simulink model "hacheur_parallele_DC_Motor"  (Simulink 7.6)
settings: Solver=ode23tb  StartTime=0.0  StopTime=500  RelTol=1e-3
InitFcn:
  | clc
  | R1=1e3;
  | R2=1e3;
StopFcn:
  | clc
  | close all
  | load vit_pos.mat
  | plotyy(x(1,:),x(2,:),x(1,:),x(3,:))
  | xlabel('temps')
  | title('position et vitesse de rotation')
  | grid
  | 
  | figure
  | 
  | load Us_CdePWM.mat
  | plotyy(y(1,:),y(2,:),y(1,:),y(3,:))
  | xlabel('temps')
  | title('Entrée PWM et tension de sortie du hâcheur parallèle')
  | grid
  | 
  | delete *.mat
libraries: fl_lib x23, powerlib x11, nesl_utility x10, elec_lib x5

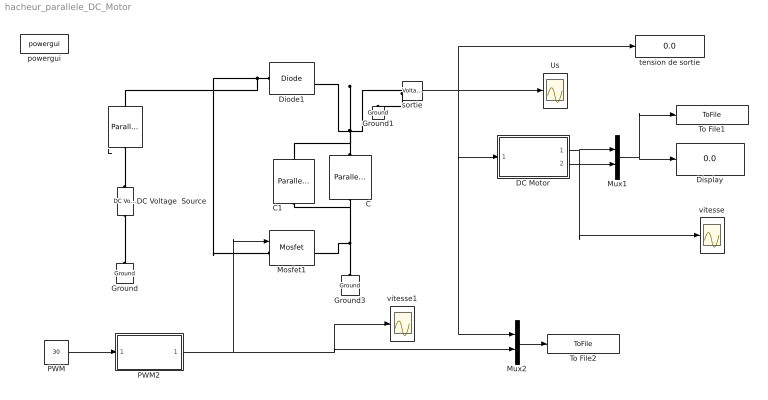
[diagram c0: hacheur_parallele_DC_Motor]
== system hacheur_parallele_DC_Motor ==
  C : powerlib/Elements/Parallel RLC Branch  DialogController=POWERSYS.PowerSysDialog  PhysicalDomain=powersysdomain  SubClassName=unknown  LeftPortType=p1  RightPortType=p1  LConnTagsString=a  RConnTagsString=__new0  BranchType=C  Resistance=1  Inductance=1e-3  SetiL0=off  InitialCurrent=0  Capacitance=1  Setx0=off  InitialVoltage=0  Measurements=None
  C1 : powerlib/Elements/Parallel RLC Branch  DialogController=POWERSYS.PowerSysDialog  PhysicalDomain=powersysdomain  SubClassName=unknown  LeftPortType=p1  RightPortType=p1  LConnTagsString=a  RConnTagsString=__new0  BranchType=C  Resistance=1  Inductance=1e-3  SetiL0=off  InitialCurrent=0  Capacitance=1  Setx0=off  InitialVoltage=0  Measurements=None
  DC Motor : Subsystem
  DC Voltage  Source : powerlib/Electrical Sources/DC Voltage Source  DialogController=POWERSYS.PowerSysDialog  SystemSampleTime=-1  Amplitude=12  Measurements=None
  Diode1 : powerlib/Power Electronics/Diode  DialogController=POWERSYS.PowerSysDialog  SystemSampleTime=-1  Ron=0.001  Lon=0  Vf=0.8  IC=0  UseSnubber=off  Rs=500  Cs=250e-9  Measurements=on
  Display : Display
  Ground : powerlib/Elements/Ground  DialogController=POWERSYS.PowerSysDialog  PhysicalDomain=powersysdomain  SubClassName=unknown  LeftPortType=p1  RightPortType=p1  LConnTagsString=a
  Ground1 : powerlib/Elements/Ground  DialogController=POWERSYS.PowerSysDialog  PhysicalDomain=powersysdomain  SubClassName=unknown  LeftPortType=p1  RightPortType=p1  LConnTagsString=a
  Ground3 : powerlib/Elements/Ground  DialogController=POWERSYS.PowerSysDialog  PhysicalDomain=powersysdomain  SubClassName=unknown  LeftPortType=p1  RightPortType=p1  LConnTagsString=a
  L : powerlib/Elements/Parallel RLC Branch  DialogController=POWERSYS.PowerSysDialog  PhysicalDomain=powersysdomain  SubClassName=unknown  LeftPortType=p1  RightPortType=p1  LConnTagsString=a  RConnTagsString=__new0  BranchType=L  Resistance=50  Inductance=1  SetiL0=off  InitialCurrent=0  Capacitance=25e-06  Setx0=off  InitialVoltage=0  Measurements=Branch voltage and current
  Mosfet1 : powerlib/Power Electronics/Mosfet  DialogController=POWERSYS.PowerSysDialog  SystemSampleTime=-1  Ron=0.1  Lon=0  Rd=0.01  Vfd=0  IC=0  Rs=1e5  Cs=inf  Measurements=on
  Mux1 : Mux  Inputs=2
  Mux2 : Mux  Inputs=2
  PWM : Constant  Value=30
  PWM2 : Subsystem
  To File1 : ToFile  Filename=vit_pos  MatrixName=x
  To File2 : ToFile  Filename=Us_CdePWM  MatrixName=y
  Us : Scope
  powergui : powerlib/powergui  SystemSampleTime=-1  SimulationMode=Continuous  SampleTime=1e-6  frequency=60  SPID=off  DisableSnubberDevices=off  DisableRonSwitches=off  DisableVfSwitches=off  SwTol=0  Interpol=off  frequencyindice=0  echomessages=off  HookPort=off  DisplayEquations=off  FunctionMessages=off  EnableUseOfTLC=off  x0status=blocks  RestoreLinks=warning  ResistiveCurrentMeasurement=off  Frange=[0:2:500]  Ylog=off  Xlog=on  ShowGrid=off  save=off  variable=ZData  ZoomFFT=on  StartTime=0.0  cycles=1  DisplayStyle=1  fundamental=60  FreqAxis=off  MaxFrequency=1000  frequencyindicesteady=1  RmsSteady=1  display=off  Ts=0  methode=off
  sortie : powerlib/Measurements/Voltage Measurement  DialogController=POWERSYS.PowerSysDialog  SystemSampleTime=-1  PhasorSimulation=off  OutputType=Complex  PSBequivalent=0
  tension de sortie : Display
  vitesse : Scope
  vitesse1 : Scope
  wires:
  sortie/1 -> Us/1, tension de sortie/1, DC Motor/1(U_induit), Mux2/1
  PWM2/1(PWM) -> Mosfet1/1, Mux2/2, vitesse1/1
  DC Motor/1(w) -> Mux1/1, vitesse/1
  DC Motor/2(alpha) -> Mux1/2
  Mux1/1 -> Display/1, To File1/1
  PWM/1 -> PWM2/1(rc (%))
  Mux2/1 -> To File2/1
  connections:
  DC Voltage  Source/LConn1 -- Ground/LConn1
  sortie/LConn1 -- Diode1/RConn1 -- C/RConn1 -- C1/RConn1
  sortie/LConn2 -- Ground1/LConn1
  L/RConn1 -- DC Voltage  Source/RConn1
  Diode1/LConn1 -- L/LConn1 -- Mosfet1/LConn1
  C/LConn1 -- Ground3/LConn1 -- Mosfet1/RConn1 -- C1/LConn1

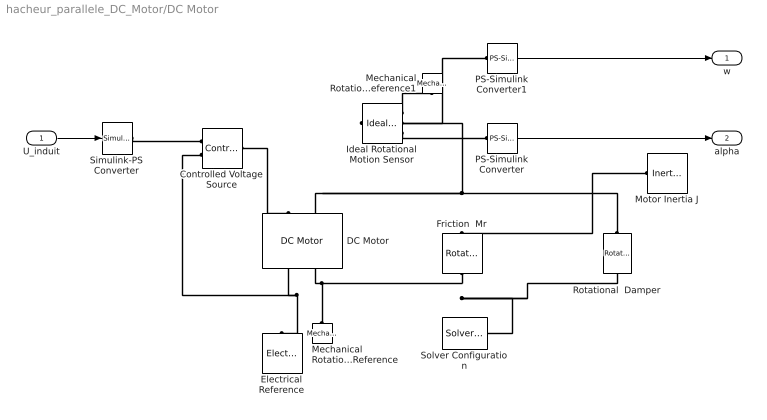
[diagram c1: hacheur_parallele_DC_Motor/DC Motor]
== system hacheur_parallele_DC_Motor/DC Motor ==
  U_induit : Inport
  Controlled Voltage Source : fl_lib/Electrical/Electrical Sources/Controlled Voltage Source  DialogController=NetworkEngine.DynNeDlgSource  SystemSampleTime=-1  i_Log=off  v_Log=off  LocalVarNames=|i|v  LocalVarDescs=|i|v  LocalVarLogging=[0 0]
  DC Motor : elec_lib/Actuators & Drivers/Rotational Actuators/DC Motor  DialogController=NetworkEngine.DynNeDlgSource  SystemSampleTime=-1  parameterization=1  Ra=3.9 Ohm  La=1.2e-3 H  emf_or_torque=2  Kv=7.2e-5 V/rpm  Ki=10e-3 N*m/A  T_stall=2.4e-4 N*m  w_max=1.91e+4 rpm  w_rated=1.5e+4 rpm  P_rated=0.08 W  V_rated=1.5 V  J=0.01 g*cm^2  lam=1e-8 N*m/(rad/s)  speed0=0 rpm  current_Log=off  voltage_Log=off  power_Log=off  i2r_Log=off  torque_Log=off  speed_Log=off  LocalVarNames=|current|voltage|power|i2r|torque|speed  LocalVarDescs=|Current (A)|Voltage (V)|Power (W)|Electrical losses (W)|Torque (Nm)|Angular speed (rad/s)  LocalVarLogging=[0 0 0 0 0 0]
  Electrical Reference : fl_lib/Electrical/Electrical Elements/Electrical Reference  DialogController=NetworkEngine.DynNeDlgSource  SystemSampleTime=-1  i_Log=off  LocalVarNames=|i  LocalVarDescs=|i  LocalVarLogging=0
  Friction  Mr : fl_lib/Mechanical/Rotational Elements/Rotational Friction  DialogController=NetworkEngine.DynNeDlgSource  SystemSampleTime=-1  brkwy_trq=0.01e-3 N*m  Col_trq=0.01e-3 N*m  visc_coef=0.001e-3 N*m/(rad/s)  trans_coef=10 s/rad  vel_thr=0.1 rad/s  t_Log=off  w_Log=off  LocalVarNames=|friction_torque|rel_velocity|power  LocalVarDescs=|Friction torque (N*m)|Relative velocity (rad/s)|Power (W)  LocalVarLogging=[0 0 0]
  Ideal Rotational Motion Sensor : fl_lib/Mechanical/Mechanical Sensors/Ideal Rotational Motion Sensor  DialogController=NetworkEngine.DynNeDlgSource  SystemSampleTime=-1  offset=0 rad  w_Log=off  t_Log=off  phi_Log=off  LocalVarNames=|w|t|phi  LocalVarDescs=|w|t|phi  LocalVarLogging=[0 0 0]
  Mechanical Rotational Reference : fl_lib/Mechanical/Rotational Elements/Mechanical Rotational Reference  DialogController=NetworkEngine.DynNeDlgSource  SystemSampleTime=-1  t_Log=off  LocalVarNames=|t  LocalVarDescs=|t  LocalVarLogging=0
  Mechanical Rotational Reference1 : fl_lib/Mechanical/Rotational Elements/Mechanical Rotational Reference  DialogController=NetworkEngine.DynNeDlgSource  SystemSampleTime=-1  t_Log=off  LocalVarNames=|t  LocalVarDescs=|t  LocalVarLogging=0
  Motor Inertia J : fl_lib/Mechanical/Rotational Elements/Inertia  DialogController=NetworkEngine.DynNeDlgSource  SystemSampleTime=-1  inertia=0.01 g*cm^2  initial_velocity=0 rad/s  t_Log=off  LocalVarNames=|torque|velocity  LocalVarDescs=|Inertia torque (N*m)|Inertia absolute velocity (rad/s)  LocalVarLogging=[0 0]
  PS-Simulink Converter : nesl_utility/PS-Simulink Converter  DialogController=NetworkEngine.DynNeUtilDlgSource  SystemSampleTime=-1  PhysicalDomain=network_engine_domain  LeftPortType=input  RightPortType=output  SubClassName=ps_output  Unit=1  AffineConversion=off
  PS-Simulink Converter1 : nesl_utility/PS-Simulink Converter  DialogController=NetworkEngine.DynNeUtilDlgSource  SystemSampleTime=-1  PhysicalDomain=network_engine_domain  LeftPortType=input  RightPortType=output  SubClassName=ps_output  Unit=1  AffineConversion=off
  Rotational  Damper : fl_lib/Mechanical/Rotational Elements/Rotational Damper  DialogController=NetworkEngine.DynNeDlgSource  SystemSampleTime=-1  D=0.01 N*m/(rad/s)  t_Log=off  w_Log=off  LocalVarNames=|t|w  LocalVarDescs=|t|w  LocalVarLogging=[0 0]
  Simulink-PS Converter : nesl_utility/Simulink-PS Converter  DialogController=NetworkEngine.DynNeUtilDlgSource  SystemSampleTime=-1  PhysicalDomain=network_engine_domain  LeftPortType=input  RightPortType=output  SubClassName=ps_input  Unit=1  AffineConversion=off  InputFilterTimeConstant=.001  UdotUserProvided=0
  Solver Configuration : nesl_utility/Solver Configuration  DialogController=NetworkEngine.DynNeUtilDlgSource  SystemSampleTime=-1  PhysicalDomain=network_engine_domain  LeftPortType=input  RightPortType=generic  SubClassName=solver  Accelerate=off  Profile=off  ResidualTolerance=1e-9  MaxNonlinIter=3  MaxModeIter=2  DoFixedCost=off  UseLocalSampling=off  DoDC=off  LinearAlgebra=Sparse  LocalSolverSampleTime=.001  LocalSolverChoice=NE_BACKWARD_EULER_ADVANCER  UseLocalSolver=off
  w : Outport
  alpha : Outport  Port=2
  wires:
  PS-Simulink Converter1/1 -> w/1
  PS-Simulink Converter/1 -> alpha/1
  U_induit/1 -> Simulink-PS Converter/1
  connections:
  Controlled Voltage Source/LConn1 -- DC Motor/LConn1
  Simulink-PS Converter/RConn1 -- Controlled Voltage Source/RConn1
  Controlled Voltage Source/RConn2 -- DC Motor/RConn1 -- Electrical Reference/LConn1
  DC Motor/LConn2 -- Ideal Rotational Motion Sensor/LConn1 -- Friction  Mr/LConn1 -- Rotational  Damper/LConn1 -- Motor Inertia J/LConn1
  Friction  Mr/RConn1 -- DC Motor/RConn2 -- Mechanical Rotational Reference/LConn1 -- Rotational  Damper/RConn1 -- Solver Configuration/RConn1
  Ideal Rotational Motion Sensor/RConn1 -- Mechanical Rotational Reference1/LConn1
  Ideal Rotational Motion Sensor/RConn2 -- PS-Simulink Converter1/LConn1
  Ideal Rotational Motion Sensor/RConn3 -- PS-Simulink Converter/LConn1

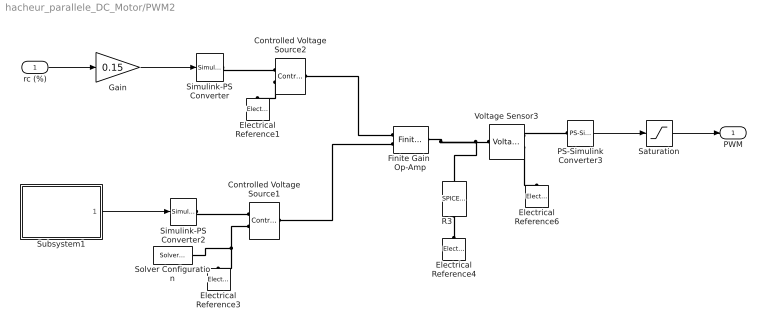
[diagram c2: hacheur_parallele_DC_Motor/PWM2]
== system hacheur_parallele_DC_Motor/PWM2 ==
  rc (%) : Inport
  Controlled Voltage Source1 : fl_lib/Electrical/Electrical Sources/Controlled Voltage Source  DialogController=NetworkEngine.DynNeDlgSource  SystemSampleTime=-1  i_Log=off  v_Log=off  LocalVarNames=|current|voltage|power  LocalVarDescs=|Current (A)|Voltage (V)|Power (W)  LocalVarLogging=[0 0 0]
  Controlled Voltage Source2 : fl_lib/Electrical/Electrical Sources/Controlled Voltage Source  DialogController=NetworkEngine.DynNeDlgSource  SystemSampleTime=-1  i_Log=off  v_Log=off  LocalVarNames=|current|voltage|power  LocalVarDescs=|Current (A)|Voltage (V)|Power (W)  LocalVarLogging=[0 0 0]
  Electrical Reference{1,3..4,6} (4 alike) : fl_lib/Electrical/Electrical Elements/Electrical Reference  DialogController=NetworkEngine.DynNeDlgSource  SystemSampleTime=-1  i_Log=off  LocalVarNames=|i  LocalVarDescs=|i  LocalVarLogging=[]
  Finite Gain  Op-Amp : elec_lib/Integrated Circuits/Finite Gain Op-Amp  DialogController=NetworkEngine.DynNeDlgSource  SystemSampleTime=-1  A=1000  Rin=1e+06 Ohm  Rout=100 Ohm  Vmin=-12 V  Vmax=12 V  LocalVarNames=|power  LocalVarDescs=|Dissipated power (W)  LocalVarLogging=0
  Gain : Gain  Gain=0.15
  PS-Simulink Converter3 : nesl_utility/PS-Simulink Converter  DialogController=NetworkEngine.DynNeUtilDlgSource  SystemSampleTime=-1  PhysicalDomain=network_engine_domain  LeftPortType=input  RightPortType=output  SubClassName=ps_output  Unit=1  AffineConversion=off
  R3 : elec_lib/Additional Components/SPICE-Compatible Components/Passive Devices/SPICE Resistor  DialogController=NetworkEngine.DynNeDlgSource  SystemSampleTime=-1  SCALE=1  R_param=1  R=10e3 Ohm  RSH=0 Ohm  LENGTH=1e-06 m  WIDTH=1e-06 m  NARROW=0 m  T_param=1  TC1=0 1/K  TC2=0 1/K^2  TOFFSET=0 K  TFIXED=300.15 K  TMEAS=300.15 K  LocalVarLogging=[]
  Saturation : Saturate  UpperLimit=1  LowerLimit=0
  Simulink-PS Converter : nesl_utility/Simulink-PS Converter  DialogController=NetworkEngine.DynNeUtilDlgSource  SystemSampleTime=-1  PhysicalDomain=network_engine_domain  LeftPortType=input  RightPortType=output  SubClassName=ps_input  Unit=1  AffineConversion=off  InputFilterTimeConstant=.001  UdotUserProvided=0
  Simulink-PS Converter2 : nesl_utility/Simulink-PS Converter  DialogController=NetworkEngine.DynNeUtilDlgSource  SystemSampleTime=-1  PhysicalDomain=network_engine_domain  LeftPortType=input  RightPortType=output  SubClassName=ps_input  Unit=1  AffineConversion=off  InputFilterTimeConstant=.001  UdotUserProvided=0
  Solver Configuration : nesl_utility/Solver Configuration  DialogController=NetworkEngine.DynNeUtilDlgSource  SystemSampleTime=-1  PhysicalDomain=network_engine_domain  LeftPortType=input  RightPortType=generic  SubClassName=solver  Accelerate=off  Profile=off  ResidualTolerance=1e-12  MaxNonlinIter=12  MaxModeIter=2  DoFixedCost=on  UseLocalSampling=off  DoDC=off  LinearAlgebra=Sparse  LocalSolverSampleTime=.001  LocalSolverChoice=NE_BACKWARD_EULER_ADVANCER  UseLocalSolver=off
  Subsystem1 : Subsystem
  Voltage Sensor3 : fl_lib/Electrical/Electrical Sensors/Voltage Sensor  DialogController=NetworkEngine.DynNeDlgSource  SystemSampleTime=-1  i1_Log=off  v1_Log=off  LocalVarNames=|i1|v1  LocalVarDescs=|i1|v1  LocalVarLogging=[]
  PWM : Outport
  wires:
  Subsystem1/1(tri) -> Simulink-PS Converter2/1
  rc (%)/1 -> Gain/1
  PS-Simulink Converter3/1 -> Saturation/1
  Saturation/1 -> PWM/1
  Gain/1 -> Simulink-PS Converter/1
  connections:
  Controlled Voltage Source1/LConn1 -- Finite Gain  Op-Amp/LConn2
  Simulink-PS Converter2/RConn1 -- Controlled Voltage Source1/RConn1
  Controlled Voltage Source1/RConn2 -- Electrical Reference3/LConn1 -- Solver Configuration/RConn1
  Finite Gain  Op-Amp/LConn1 -- Controlled Voltage Source2/LConn1
  Simulink-PS Converter/RConn1 -- Controlled Voltage Source2/RConn1
  Controlled Voltage Source2/RConn2 -- Electrical Reference1/LConn1
  Electrical Reference4/LConn1 -- R3/LConn1
  Voltage Sensor3/RConn2 -- Electrical Reference6/LConn1
  Finite Gain  Op-Amp/RConn1 -- R3/RConn1 -- Voltage Sensor3/LConn1
  Voltage Sensor3/RConn1 -- PS-Simulink Converter3/LConn1

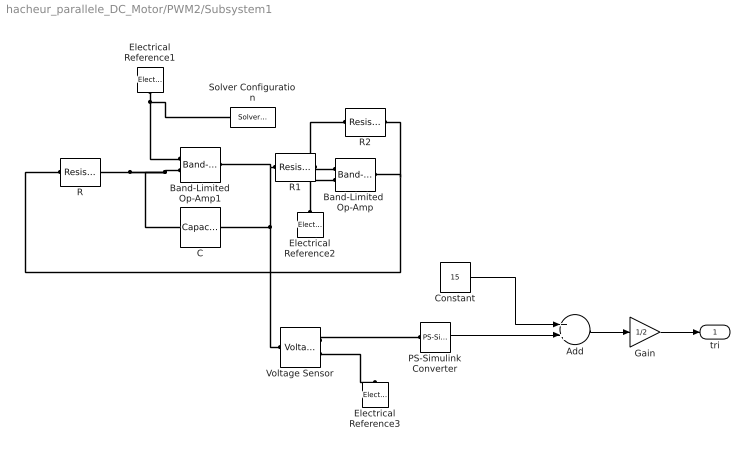
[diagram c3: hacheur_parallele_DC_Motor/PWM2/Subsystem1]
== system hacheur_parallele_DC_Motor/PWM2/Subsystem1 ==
  Add : Sum
  Band-Limited  Op-Amp : elec_lib/Integrated Circuits/Band-Limited Op-Amp  DialogController=NetworkEngine.DynNeDlgSource  SystemSampleTime=-1  A=1000  Rin=1e+06 Ohm  Rout=100 Ohm  Vmin=-15 V  Vmax=15 V  Vdotmax=1000 V/s  f=1e+05 Hz  V0=0 V  LocalVarNames=|power  LocalVarDescs=|Dissipated power (W)  LocalVarLogging=0
  Band-Limited Op-Amp1 : elec_lib/Integrated Circuits/Band-Limited Op-Amp  DialogController=NetworkEngine.DynNeDlgSource  SystemSampleTime=-1  A=1000  Rin=1e+06 Ohm  Rout=100 Ohm  Vmin=-15 V  Vmax=15 V  Vdotmax=1000 V/s  f=1e+05 Hz  V0=0 V  LocalVarNames=|power  LocalVarDescs=|Dissipated power (W)  LocalVarLogging=0
  C : fl_lib/Electrical/Electrical Elements/Capacitor  DialogController=NetworkEngine.DynNeDlgSource  SystemSampleTime=-1  c=0.1e-5 F  v0=0.1 V  r=1e-6 Ohm  g=0 1/Ohm  i_Log=off  v_Log=off  vc_Log=off  LocalVarNames=|current|voltage|power  LocalVarDescs=|Capacitor current (A)|Voltage across capacitor (V)|Power (W)  LocalVarLogging=[0 0 0]
  Constant : Constant  Value=15
  Electrical Reference1 : fl_lib/Electrical/Electrical Elements/Electrical Reference  DialogController=NetworkEngine.DynNeDlgSource  SystemSampleTime=-1  i_Log=off  LocalVarNames=|i  LocalVarDescs=|i  LocalVarLogging=[]
  Electrical Reference2 : fl_lib/Electrical/Electrical Elements/Electrical Reference  DialogController=NetworkEngine.DynNeDlgSource  SystemSampleTime=-1  i_Log=off  LocalVarNames=|i  LocalVarDescs=|i  LocalVarLogging=[]
  Electrical Reference3 : fl_lib/Electrical/Electrical Elements/Electrical Reference  DialogController=NetworkEngine.DynNeDlgSource  SystemSampleTime=-1  i_Log=off  LocalVarNames=|i  LocalVarDescs=|i  LocalVarLogging=[]
  Gain : Gain  Gain=1/2
  PS-Simulink Converter : nesl_utility/PS-Simulink Converter  DialogController=NetworkEngine.DynNeUtilDlgSource  SystemSampleTime=-1  PhysicalDomain=network_engine_domain  LeftPortType=input  RightPortType=output  SubClassName=ps_output  Unit=1  AffineConversion=off
  R : fl_lib/Electrical/Electrical Elements/Resistor  DialogController=NetworkEngine.DynNeDlgSource  SystemSampleTime=-1  R=1000 Ohm  i_Log=off  v_Log=off  LocalVarNames=|current|voltage|power  LocalVarDescs=|Resistor current (A)|Voltage across resistor (V)|Power (W)  LocalVarLogging=[0 0 0]
  R1 : fl_lib/Electrical/Electrical Elements/Resistor  DialogController=NetworkEngine.DynNeDlgSource  SystemSampleTime=-1  R=10e3 Ohm  i_Log=off  v_Log=off  LocalVarNames=|current|voltage|power  LocalVarDescs=|Resistor current (A)|Voltage across resistor (V)|Power (W)  LocalVarLogging=[0 0 0]
  R2 : fl_lib/Electrical/Electrical Elements/Resistor  DialogController=NetworkEngine.DynNeDlgSource  SystemSampleTime=-1  R=10e3 Ohm  i_Log=off  v_Log=off  LocalVarNames=|current|voltage|power  LocalVarDescs=|Resistor current (A)|Voltage across resistor (V)|Power (W)  LocalVarLogging=[0 0 0]
  Solver Configuration : nesl_utility/Solver Configuration  DialogController=NetworkEngine.DynNeUtilDlgSource  SystemSampleTime=-1  PhysicalDomain=network_engine_domain  LeftPortType=input  RightPortType=generic  SubClassName=solver  Accelerate=off  Profile=off  ResidualTolerance=1e-9  MaxNonlinIter=12  MaxModeIter=2  DoFixedCost=off  UseLocalSampling=off  DoDC=off  LinearAlgebra=Sparse  LocalSolverSampleTime=.001  LocalSolverChoice=NE_BACKWARD_EULER_ADVANCER  UseLocalSolver=off
  Voltage Sensor : fl_lib/Electrical/Electrical Sensors/Voltage Sensor  DialogController=NetworkEngine.DynNeDlgSource  SystemSampleTime=-1  i1_Log=off  v1_Log=off  LocalVarNames=|i1|v1  LocalVarDescs=|i1|v1  LocalVarLogging=[]
  tri : Outport
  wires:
  Gain/1 -> tri/1
  Add/1 -> Gain/1
  Constant/1 -> Add/1
  PS-Simulink Converter/1 -> Add/2
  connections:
  Voltage Sensor/RConn2 -- Electrical Reference3/LConn1
  R1/RConn1 -- Band-Limited  Op-Amp/LConn1 -- R2/LConn1
  Electrical Reference2/LConn1 -- Band-Limited  Op-Amp/LConn2
  R2/RConn1 -- Band-Limited  Op-Amp/RConn1 -- R/LConn1
  Electrical Reference1/LConn1 -- Band-Limited Op-Amp1/LConn1 -- Solver Configuration/RConn1
  Band-Limited Op-Amp1/LConn2 -- C/LConn1 -- R/RConn1
  Voltage Sensor/LConn1 -- C/RConn1 -- R1/LConn1 -- Band-Limited Op-Amp1/RConn1
  Voltage Sensor/RConn1 -- PS-Simulink Converter/LConn1
